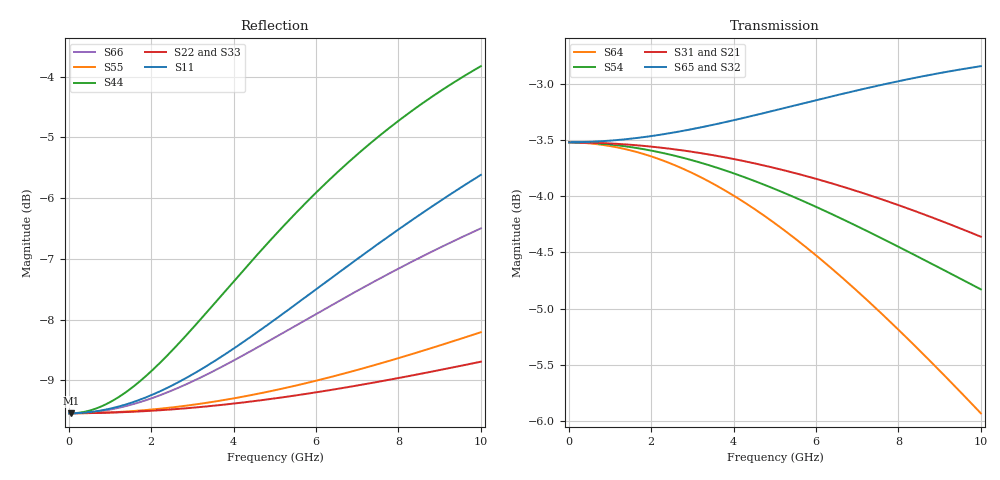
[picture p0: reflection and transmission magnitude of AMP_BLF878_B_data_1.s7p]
! Created Wed Mar 10 14:50:47 2010
# ghz S ma R 50
! 7 Port Network Data from SP1.SP block
! freq  magS11  angS11  magS12  angS12  magS13  angS13  magS14  angS14
!  magS15  angS15  magS16  angS16  magS17  angS17
!  magS21  angS21
!  magS22  angS22  magS23  angS23  magS24  angS24  magS25  angS25
!  magS26  angS26  magS27  angS27
!  magS31  angS31  magS32  angS32
!  magS33  angS33  magS34  angS34  magS35  angS35  magS36  angS36
!  magS37  angS37
!  magS41  angS41  magS42  angS42  magS43  angS43
!  magS44  angS44  magS45  angS45  magS46  angS46  magS47  angS47
!  magS51  angS51  magS52  angS52  magS53  angS53  magS54  angS54
!  magS55  angS55  magS56  angS56  magS57  angS57
!  magS61  angS61
!  magS62  angS62  magS63  angS63  magS64  angS64  magS65  angS65
!  magS66  angS66  magS67  angS67
!  magS71  angS71  magS72  angS72
!  magS73  angS73  magS74  angS74  magS75  angS75  magS76  angS76
!  magS77  angS77
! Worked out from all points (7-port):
!   1000 points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, 10 MHz to 10 GHz, reference 50 ohm
!   strongest paths, dB at 10 MHz, 2.51 GHz, 5.01 GHz, 7.51 GHz, 10 GHz:
!     S65: -3.5, -3.4, -3.2, -3.0, -2.8
!     S32: -3.5, -3.5, -3.3, -3.2, -3.0
!     S31: -3.5, -3.6, -3.8, -4.0, -4.4
!     S21: -3.5, -3.6, -3.8, -4.1, -4.5
!     S54: -3.5, -3.6, -3.9, -4.4, -4.8
!     S64: -3.5, -3.7, -4.2, -5.0, -5.9
!   lowest |S11| = -9.5 dB at 50 MHz (marker M1), VSWR 2.00, Z = 25 + j0.179 ohm
!   |S11| at or under -10 dB: nowhere
